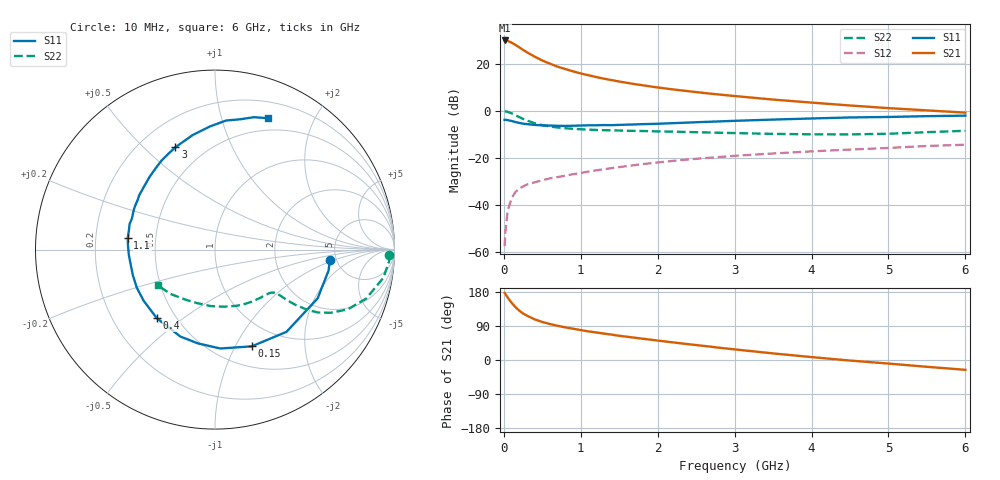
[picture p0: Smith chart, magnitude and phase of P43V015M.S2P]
! SIEMENS Small Signal Semiconductors
! BFP182
! Si NPN RF Bipolar Junction Transistor in SOT143
! VCE = 3 V  IC = 15 mA
! Common Emitter S-Parameters:  March  1996
# GHz  S  MA  R  50
!  f  S11  S21  S12  S22
! GHz  MAG  ANG  MAG  ANG  MAG  ANG  MAG  ANG
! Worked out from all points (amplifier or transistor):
!   36 points, 10 MHz to 6 GHz, reference 50 ohm
!   highest |S21| = 30.0 dB at 10 MHz (marker M1)
!   |S21| within 3 dB of that: start of sweep to 203.8 MHz
!   unconditionally stable (mu >= 1): 914.5 MHz to 5.322 GHz
!   at 250 MHz: K = 0.42, MSG = 29.1 dB, |S12| = -32.3 dB
!   at 1.4 GHz: K = 1.14, MAG = 16.5 dB, |S12| = -24.5 dB
!   at 6 GHz: K = 0.92, MSG = 6.8 dB, |S12| = -14.5 dB
!   S11 on the Smith chart (normalised r, x): 10 MHz: 4.42, -0.86; 150 MHz: 0.72, -1.17; 400 MHz: 0.39, -0.40; 1.1 GHz: 0.34, +0.06; 3 GHz: 0.34, +0.63; 6 GHz: 0.36, +1.42
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0.01  0.6424 -5.1  31.64 177.0  0.0013 87.1  0.9722 -1.7
0.02  0.6436 -10.4  31.62 174.1  0.0026 85.6  0.9722 -3.9
0.05  0.6331 -25.4  31.04 164.8  0.0074 84.5  0.9505 -9.6
0.1  0.6071 -49.0  28.43 151.2  0.0136 67.6  0.8849 -18.0
0.15  0.5765 -69.2  25.48 139.7  0.0185 61.2  0.8113 -24.2
0.2  0.5519 -86.9  22.62 130.2  0.022 56.3  0.7355 -28.6
0.25  0.531 -100.5  19.91 122.8  0.0244 54.2  0.6727 -31.4
0.3  0.5213 -111.8  17.75 117.1  0.0268 51.1  0.62 -33.0
0.4  0.5011 -130.4  14.31 107.3  0.0299 49.1  0.5437 -34.5
0.5  0.4892 -144.3  11.81 100.3  0.0331 47.2  0.4946 -35.0
0.6  0.4847 -154.0  10.13 94.9  0.0363 47.9  0.4631 -35.1
0.7  0.4794 -162.7  8.731 90.2  0.0387 49.0  0.4405 -35.2
0.9  0.4809 -176.4  6.946 82.5  0.0446 49.9  0.4124 -35.7
1.1  0.4907 172.4  5.732 75.5  0.0507 50.4  0.3967 -37.2
1.5  0.5011 155.4  4.215 63.9  0.0631 50.5  0.38 -41.4
1.8  0.5195 144.4  3.511 56.2  0.0729 49.7  0.3707 -45.7
2.2  0.5453 131.9  2.857 46.4  0.0856 47.3  0.3595 -52.4
3  0.6116 111.1  2.067 28.0  0.1097 41.4  0.3354 -69.0
3.5  0.6503 101.0  1.736 17.4  0.1231 37.2  0.3221 -81.1
4.5  0.7218 85.1  1.299 -1.5  0.1492 29.0  0.3145 -108.2
5.5  0.769 73.6  1.022 -18.0  0.1778 21.2  0.3502 -135.2
6  0.7892 68.1  0.914 -25.9  0.1892 16.3  0.3753 -147.9
